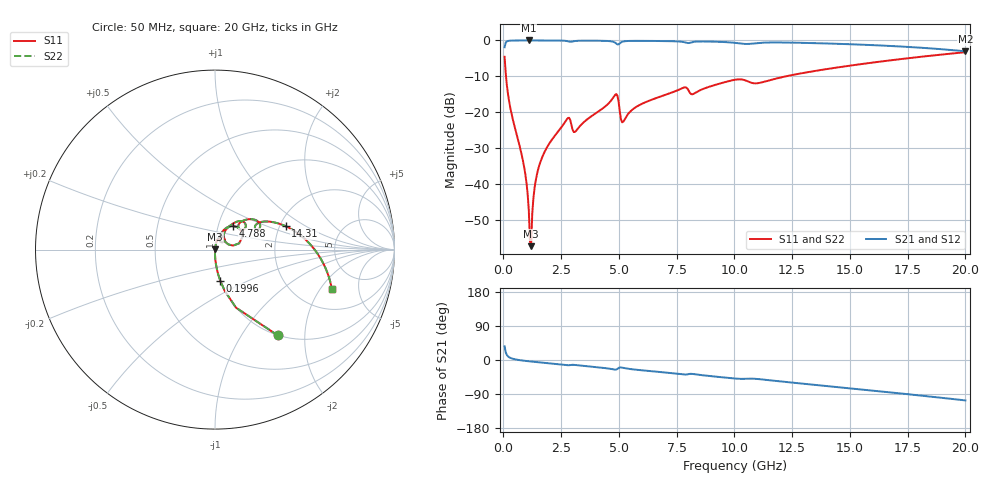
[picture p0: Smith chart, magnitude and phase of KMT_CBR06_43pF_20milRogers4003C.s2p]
! Data measured by Modelithics Inc. support@modelithics.com 813-866-6335
! KEMET CBR0603 43pF, Pad Width= 0.851mm, Pad Length= 0.64mm, Pad Gap= 0.62mm, 20mil Rogers 4003C substrate Data, January 2022
# hz S ma R 50
! 2 Port Network Data from SP1.SP block
! freq  magS11  angS11  magS21  angS21  magS12  angS12  magS22  angS22
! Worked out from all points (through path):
!   401 points, 50 MHz to 20 GHz, reference 50 ohm
!   highest |S21| = -0.01 dB at 1.097 GHz (marker M1); lowest = -3.0 dB at 20 GHz (marker M2)
!   group delay of S21, straight-line fit = 14.9 ps
!   lowest |S11| = -57.2 dB at 1.197 GHz (marker M3), VSWR 1.00, Z = 50.1 + j0.118 ohm
!   |S11| at or under -10 dB: 110.9 MHz to 12.22 GHz (12.11 GHz wide, 196 % of centre)
!   |S22| runs from -57.2 to -3.3 dB; largest |S21 - S12| = 0
!   S11 on the Smith chart (normalised r, x): 50 MHz: 1.00, -1.47; 199.6 MHz: 1.00, -0.36; 4.788 GHz: 1.18, +0.32; 14.31 GHz: 2.15, +0.68; 20 GHz: 3.13, -2.56
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5e7  0.5925 -53.8  0.8051 36.2  0.8051 36.2  0.5925 -53.8
1.99625e8  0.1765 -80.4  0.9839 9.5  0.9839 9.5  0.1765 -80.4
8.97875e8  0.01722 -90.2  0.9993 -2.0  0.9993 -2.0  0.01722 -90.2
9.97625e8  0.01042 -89.6  0.9993 -2.7  0.9993 -2.7  0.01042 -89.6
1.097375e9  0.00436 -85.6  0.9994 -3.4  0.9994 -3.4  0.00436 -85.6
1.197125e9  0.001378 59.1  0.9993 -4.0  0.9993 -4.0  0.001378 59.1
1.4465e9  0.01357 81.5  0.9992 -5.5  0.9992 -5.5  0.01357 81.5
1.8455e9  0.03096 80.5  0.9985 -7.9  0.9985 -7.9  0.03096 80.5
2.74325e9  0.07993 65.2  0.9812 -13.5  0.9812 -13.5  0.07993 65.2
3.092375e9  0.05326 58.0  0.9813 -13.1  0.9813 -13.1  0.05326 58.0
3.391625e9  0.06872 70.0  0.9916 -15.1  0.9916 -15.1  0.06872 70.0
4.788125e9  0.1667 51.9  0.9488 -25.1  0.9488 -25.1  0.1667 51.9
4.887875e9  0.1795 36.7  0.9026 -25.2  0.9026 -25.2  0.1795 36.7
5.187125e9  0.07401 44.3  0.9665 -20.9  0.9665 -20.9  0.07401 44.3
5.73575e9  0.1184 61.4  0.9865 -25.6  0.9865 -25.6  0.1184 61.4
6.73325e9  0.1631 57.1  0.9822 -31.4  0.9822 -31.4  0.1631 57.1
1.0025e10  0.284 34.4  0.926 -49.0  0.926 -49.0  0.284 34.4
1.10225e10  0.2546 29.3  0.9213 -50.2  0.9213 -50.2  0.2546 29.3
1.336662e10  0.3709 23.7  0.9191 -64.8  0.9191 -64.8  0.3709 23.7
1.431425e10  0.4145 18.3  0.9012 -70.5  0.9012 -70.5  0.4145 18.3
1.670825e10  0.5268 3.8  0.8395 -85.2  0.8395 -85.2  0.5268 3.8
2e10  0.6858 -18.4  0.7056 -106.6  0.7056 -106.6  0.6858 -18.4
